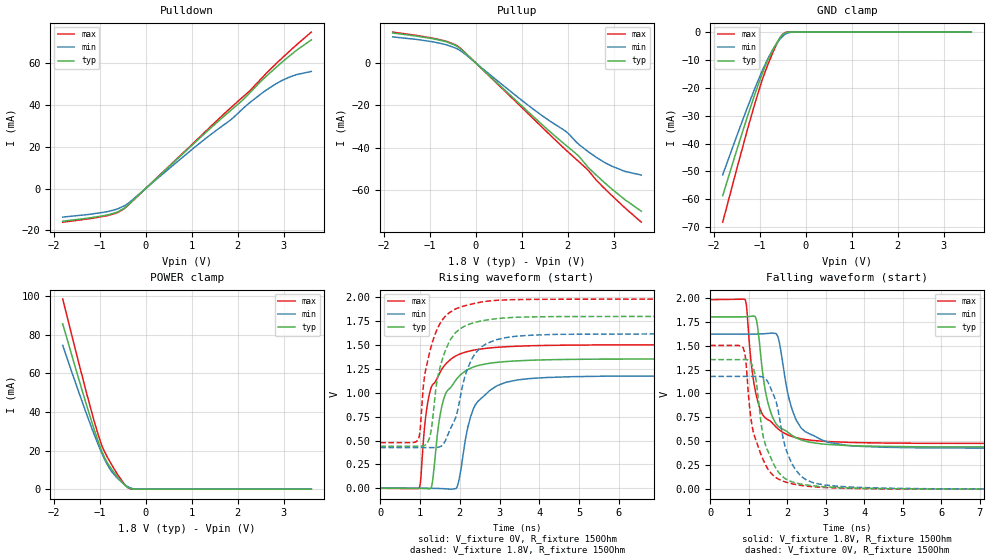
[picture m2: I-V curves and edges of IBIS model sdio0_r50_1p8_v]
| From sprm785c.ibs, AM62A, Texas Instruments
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|   r50_1p8_v
[Model]   sdio0_r50_1p8_v
Model_type   I/O
Polarity   Non-Inverting
Enable   Active-High
Vinl = 0
Vinh = 0.8
Vmeas = 0.9
Vref = 1.8
Cref = 2pF
Rref = 100000
|   typ   min   max
C_comp   6.976pF   6.800pF   6.977pF
[Voltage Range]   1.8   1.62   1.98
[Temperature Range]   27   150   -40
[Pullup Reference]   1.8   1.62   1.98
[Pulldown Reference]   0   0   0
[Power Clamp Reference]   1.8   1.62   1.98
[GND Clamp Reference]   0   0   0
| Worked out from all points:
|   slope of the pulldown table from 0 to 0.27 V, typ, clamps not added: 48.5 ohm
|   slope of the pullup table from 0 to 0.27 V, typ, clamps not added: 49.3 ohm
|   GND clamp passes 1 mA (typ) near -0.50 V on its own axis
|   POWER clamp passes 1 mA (typ) near -0.39 V on its own axis
|   falling waveform, V_fixture 1.8V, R_fixture 150Ohm: 20-80 % time 390ps typ, 461ps min, 376ps max; typ from 1.8 V to 0.44 V
|   rising waveform, V_fixture 0V, R_fixture 150Ohm: 20-80 % time 452ps typ, 501ps min, 437ps max; typ from 0 V to 1.35 V
|   rising waveform, V_fixture 1.8V, R_fixture 150Ohm: 20-80 % time 415ps typ, 530ps min, 416ps max; typ from 0.44 V to 1.8 V
|   falling waveform, V_fixture 0V, R_fixture 150Ohm: 20-80 % time 430ps typ, 481ps min, 429ps max; typ from 1.35 V to 0 V
[Pulldown]
|   Voltage   I(typ)   I(min)   I(max)
-1.8V     -15.59mA   -13.63mA   -16.08mA
-817.2mV  -12.54mA   -10.95mA   -12.85mA
-595.8mV  -11.05mA   -9.615mA   -11.36mA
-450mV    -9.164mA   -8.111mA   -9.376mA
1.364V    27.99mA    24.99mA    28.65mA
1.84V     37.22mA    32.73mA    38.47mA
2.12V     42.6mA     38.39mA    43.99mA
2.266V    45.89mA    41.18mA    46.85mA
2.612V    53.57mA    47mA       54.94mA
2.833V    57.97mA    50.16mA    59.73mA
3.098V    62.96mA    53.1mA     65.16mA
3.6V      71.18mA    56.04mA    74.89mA
[GND Clamp]
|   Voltage   I(typ)   I(min)   I(max)
-1.8V     -58.72mA   -51.23mA   -68.24mA
-1.271V   -30.69mA   -27.39mA   -35.46mA
-1.098V   -22.1mA    -20.06mA   -25.47mA
-952.2mV  -15.37mA   -14.29mA   -17.66mA
-822.6mV  -10.14mA   -9.655mA   -11.8mA
-671.4mV  -5.164mA   -5.19mA    -5.873mA
-563.4mV  -2.202mA   -2.714mA   -2.268mA
-487.8mV  -770.8uA   -1.357mA   -614.7uA
-439.2mV  -272.6uA   -734.7uA   -140.4uA
-369mV    -35.99uA   -217.7uA   -8.949uA
-255.6mV  -694.5nA   -16.47uA   -114.5nA
3.6V      0A         0A         0A
[Pullup]
|   Voltage   I(typ)   I(min)   I(max)
-1.8V     13.99mA    12.15mA    14.42mA
-887.4mV  11.14mA    9.69mA     11.39mA
-628.2mV  9.783mA    8.4mA      10.04mA
-358.2mV  7.063mA    6.037mA    7.355mA
1.138V    -22.94mA   -19.89mA   -23.81mA
1.948V    -38.5mA    -32.03mA   -40.68mA
2.201V    -43.08mA   -37.52mA   -45.66mA
2.434V    -48.84mA   -41.56mA   -50.21mA
2.612V    -52.6mA    -44.28mA   -54.89mA
2.936V    -58.88mA   -48.36mA   -61.89mA
3.222V    -63.94mA   -50.86mA   -67.72mA
3.6V      -69.75mA   -52.74mA   -74.9mA
[POWER Clamp]
|   Voltage   I(typ)   I(min)   I(max)
-1.8V     85.65mA    74.47mA    98.51mA
-1.287V   43.92mA    39.26mA    50.24mA
-1.13V    31.96mA    29.2mA     36.42mA
-1.006V   23.2mA     21.73mA    26.43mA
-892.8mV  16.49mA    15.59mA    19.51mA
-736.2mV  10.27mA    9.092mA    12.63mA
-595.8mV  5.806mA    5.297mA    7.095mA
-450mV    2.033mA    2.29mA     2.335mA
-390.6mV  941.9uA    1.376mA    958.2uA
-315mV    199.5uA    531.1uA    119.4uA
-147.6mV  836.5nA    14.06uA    186.2nA
3.6V      0A         0A         0A
[Ramp]
R_load = 150
|   typ   min   max
dV/dt_r   0.81209/4.51629e-10   0.706646/5.06979e-10   0.90074/4.37029e-10
dV/dt_f   0.815746/3.8765e-10   0.715995/4.55706e-10   0.901311/3.75736e-10
[Falling Waveform]
V_fixture = 1.8V
V_fixture_min = 1.62V
V_fixture_max = 1.98V
R_fixture = 150Ohm
C_fixture = 0F
|   Time   V(typ)   V(min)   V(max)
0s        1.8V       1.62V      1.98V
905ps     1.801V     1.62V      1.979V
1.17ns    1.8V       1.62V      1.026V
1.41ns    1.073V     1.624V     752.4mV
1.54ns    839.9mV    1.628V     716mV
1.755ns   661.1mV    1.592V     631.4mV
2.045ns   585.2mV    945.5mV    561mV
2.46ns    502.2mV    601.9mV    519.9mV
3.55ns    456.2mV    457.3mV    489.6mV
10ns      440.2mV    426.2mV    477.7mV
[Rising Waveform]
V_fixture = 0V
V_fixture_min = 0V
V_fixture_max = 0V
R_fixture = 150Ohm
C_fixture = 0F
|   Time   V(typ)   V(min)   V(max)
0s        241.8uV    537.6uV    159.3uV
980ps     -1.009mV   421.7uV    1.741mV
1.135ns   -2.888mV   483.5uV    722.4mV
1.275ns   645uV      -98.78uV   1.048V
1.58ns    910.4mV    -3.93mV    1.264V
1.92ns    1.143V     4.476mV    1.389V
2.06ns    1.202V     283.5mV    1.414V
2.39ns    1.275V     871.9mV    1.448V
3.17ns    1.326V     1.11V      1.481V
10ns      1.354V     1.178V     1.501V
[Rising Waveform]
V_fixture = 1.8V
V_fixture_min = 1.62V
V_fixture_max = 1.98V
R_fixture = 150Ohm
C_fixture = 0F
|   Time   V(typ)   V(min)   V(max)
0s        440.2mV    426.2mV    477.7mV
950ps     439.9mV    426.1mV    505.5mV
1.175ns   468.9mV    426mV      1.301V
1.27ns    582mV      425.8mV    1.468V
1.415ns   1.091V     427.9mV    1.647V
1.53ns    1.305V     440.3mV    1.743V
1.995ns   1.664V     914.2mV    1.893V
2.405ns   1.738V     1.419V     1.937V
3.165ns   1.783V     1.577V     1.971V
10ns      1.8V       1.62V      1.98V
[Falling Waveform]
|Gnd
V_fixture = 0V
V_fixture_min = 0V
V_fixture_max = 0V
R_fixture = 150Ohm
C_fixture = 0F
|   Time   V(typ)   V(min)   V(max)
0s        1.354V     1.178V     1.501V
850ps     1.354V     1.178V     1.479V
920ps     1.354V     1.178V     1.35V
1.05ns    1.327V     1.178V     753mV
1.43ns    465.9mV    1.156V     258.5mV
1.715ns   210.7mV    904.9mV    118.2mV
1.925ns   116.1mV    472mV      78.32mV
2.335ns   54.97mV    143.7mV    40.84mV
2.965ns   24.68mV    44.02mV    17.69mV
10ns      241.7uV    537.8uV    159.2uV
